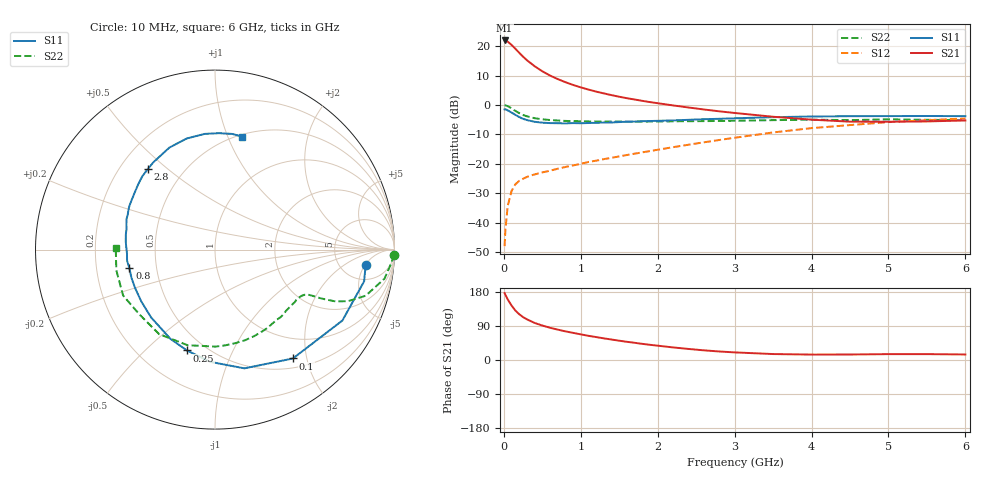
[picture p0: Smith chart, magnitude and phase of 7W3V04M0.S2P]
! Infineon Technologies  Discrete & RF Semiconductors
! BFS17W
! Si NPN RF Bipolar Junction Transistor in SOT323
! VCE = 3 V  IC = 4 mA
! Common Emitter S-Parameters:  August  1999
# GHz  S  MA  R  50
!  f  S11  S21  S12  S22
! GHz  MAG  ANG  MAG  ANG  MAG  ANG  MAG  ANG
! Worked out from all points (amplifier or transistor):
!   36 points, 10 MHz to 6 GHz, reference 50 ohm
!   highest |S21| = 22.0 dB at 10 MHz (marker M1)
!   |S21| within 3 dB of that: start of sweep to 156.5 MHz
!   unconditionally stable (mu >= 1): 599.8 MHz to 3.025 GHz; 4.114 GHz to end of sweep
!   at 250 MHz: K = 0.53, MSG = 20.7 dB, |S12| = -25.0 dB
!   at 1.4 GHz: K = 1.27, MAG = 7.5 dB, |S12| = -17.9 dB
!   at 6 GHz: K = 1.09, MAG = -2.1 dB, |S12| = -4.6 dB
!   S11 on the Smith chart (normalised r, x): 10 MHz: 9, -5; 100 MHz: 0.64, -1.76; 250 MHz: 0.40, -0.68; 800 MHz: 0.35, -0.09; 2.8 GHz: 0.31, +0.43; 6 GHz: 0.52, +1.13
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0.01  0.8438 -5.8  12.53 176.5  0.004 83.6  0.9956 -1.6
0.02  0.8495 -12.0  12.46 171.9  0.0076 83.9  0.9874 -4.0
0.05  0.8124 -29.1  11.97 160.1  0.0192 75.8  0.9584 -9.7
0.1  0.746 -54.4  10.54 143.8  0.0346 63.7  0.8782 -17.0
0.15  0.6816 -76.1  9.053 130.5  0.045 55.3  0.7949 -21.2
0.2  0.6262 -92.3  7.734 120.8  0.0515 51.0  0.7297 -23.3
0.25  0.5831 -105.6  6.643 113.2  0.056 47.3  0.6785 -24.2
0.3  0.5561 -116.4  5.784 107.3  0.0601 46.5  0.6447 -24.8
0.4  0.5194 -133.2  4.572 97.8  0.0663 45.7  0.5978 -25.4
0.5  0.5022 -144.8  3.754 91.0  0.0717 47.0  0.5729 -25.9
0.6  0.494 -154.3  3.175 85.1  0.0765 48.6  0.5572 -26.9
0.8  0.4883 -167.8  2.449 75.6  0.0887 51.4  0.5379 -30.0
0.9  0.4937 -172.9  2.196 71.6  0.0941 53.2  0.5328 -31.7
1.1  0.4953 177.9  1.833 63.8  0.1079 55.9  0.5269 -35.9
1.3  0.5041 170.1  1.578 57.1  0.1206 57.8  0.5225 -40.8
1.6  0.5217 160.8  1.307 48.0  0.1417 60.5  0.5212 -48.4
2.2  0.5487 144.7  0.986 33.2  0.1925 63.8  0.5292 -65.6
2.8  0.5843 129.9  0.783 22.5  0.2547 63.5  0.5365 -83.9
3.5  0.6226 114.1  0.633 15.7  0.3424 59.3  0.5542 -106.0
4.5  0.6472 95.1  0.522 14.5  0.457 47.4  0.5546 -139.3
5.5  0.6515 81.5  0.527 15.5  0.5533 35.0  0.5616 -168.2
6  0.6478 76.4  0.548 14.6  0.5915 28.9  0.5531 179.2
